(* Logix 5000 Routine export Unit1_Hold; software revision 20.05 *)

TYPE Unit_Type :   // Common information for a unit
STRUCT
   Alm_Reset : BOOL;   // Alarm reset
   Local : BOOL;   // Local/remote control indication
   Maint : BOOL;   // Maintenance privilege for device control
   Man_StartOpen : BOOL;   // Manual start/open from operator
   Man_StopClose : BOOL;   // Manual stop/close from operator
   Man_DevNum : DINT;   // Number of device started/stopped at OI
   Msg : DINT;   // Message number
   Time_Remaining : DINT;   // Remaining time in timed steps
END_STRUCT
END_TYPE

TYPE Seq_Type :   // Sequence Information
STRUCT
   Step_Num : DINT;   // Current step number
   Running : BOOL;   // Running indication
   PC_Start : BOOL;   // Sequence start request from PC
   LTP_Start : BOOL;   // Sequence start request from LTP
   Ons : BOOL;   // One-shot storage to start
   Auto_Start : BOOL;   // Auto-start request
   Auto_Ons : BOOL;   // Auto-start one-shot storage
   Req_Tmr : TIMER;   // Auto-start hold timer
END_STRUCT
END_TYPE

VAR_GLOBAL   (* controller tags *)
   Unit1_Hold : Seq_Type := (Req_Tmr.PRE := 5000);   // Unit Desc1 Hold Sequence
   Unit1_Sample : Seq_Type := (Req_Tmr.PRE := 5000);   // Unit Desc1 Sample Sequence
   Unit1 : Unit_Type;   // Unit Desc1
   Unit1_Shutdown : Seq_Type := (Req_Tmr.PRE := 5000);   // Unit Desc1 Shutdown Sequence
   Unit1_Eshutdown : Seq_Type := (Req_Tmr.PRE := 5000);   // Unit Desc1 E-Shutdown Sequence
END_VAR

PROGRAM MainProgram

ROUTINE Unit1_Hold   (* ladder *)
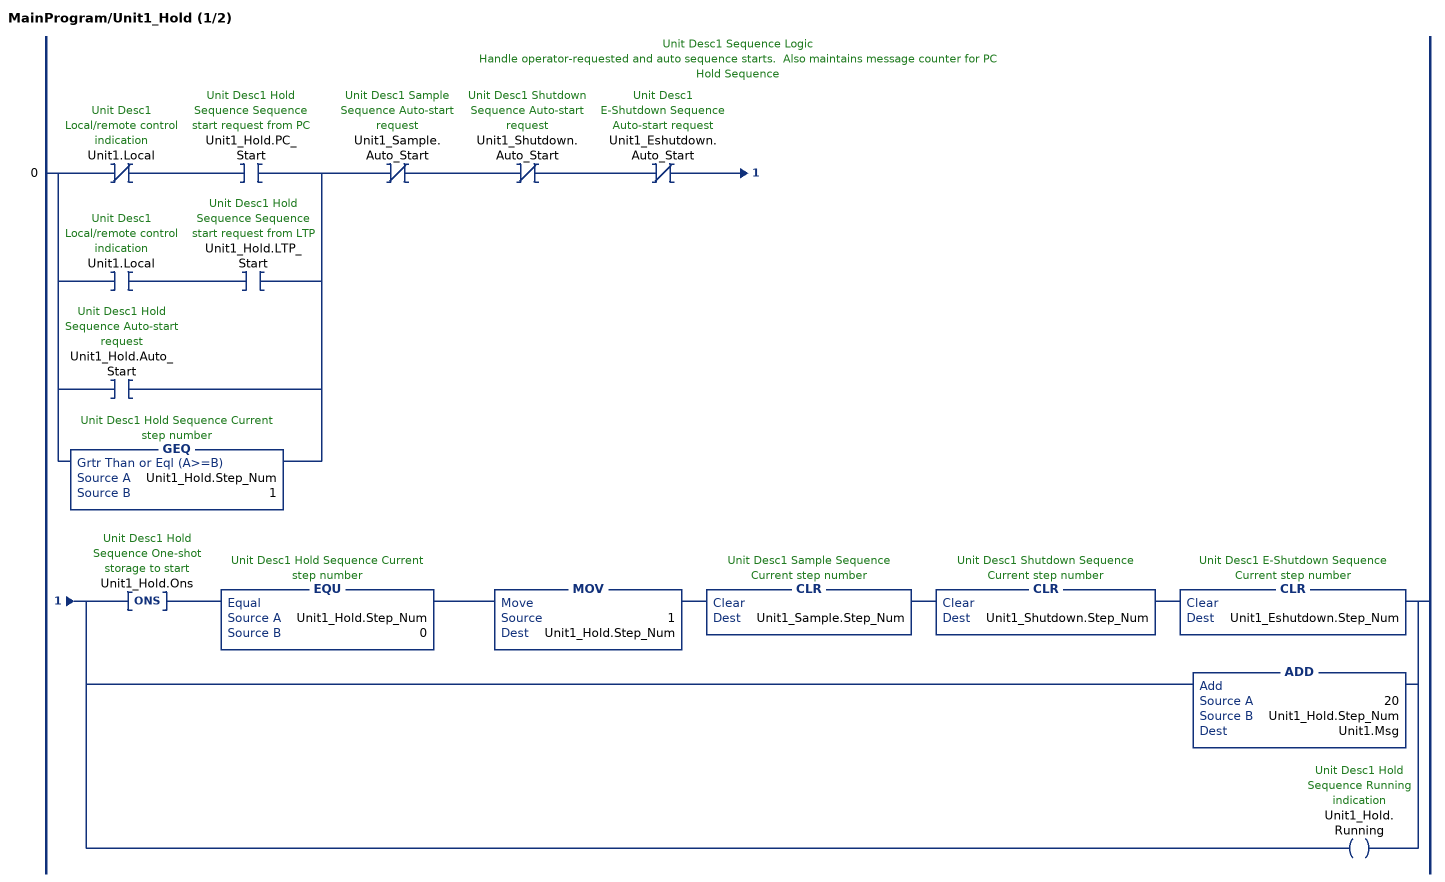
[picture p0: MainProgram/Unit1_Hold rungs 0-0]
   // Unit Desc1 Sequence Logic
   // Handle operator-requested and auto sequence starts.  Also maintains message counter for PC
   // Hold Sequence
   0: [XIO(Unit1.Local) XIC(Unit1_Hold.PC_Start) ,XIC(Unit1.Local) XIC(Unit1_Hold.LTP_Start) ,XIC(Unit1_Hold.Auto_Start) ,GEQ(Unit1_Hold.Step_Num,1) ]XIO(Unit1_Sample.Auto_Start)XIO(Unit1_Shutdown.Auto_Start)XIO(Unit1_Eshutdown.Auto_Start)[ONS(Unit1_Hold.Ons) EQU(Unit1_Hold.Step_Num,0) MOV(1,Unit1_Hold.Step_Num) CLR(Unit1_Sample.Step_Num) CLR(Unit1_Shutdown.Step_Num) CLR(Unit1_Eshutdown.Step_Num) ,ADD(20,Unit1_Hold.Step_Num,Unit1.Msg) ,OTE(Unit1_Hold.Running) ];
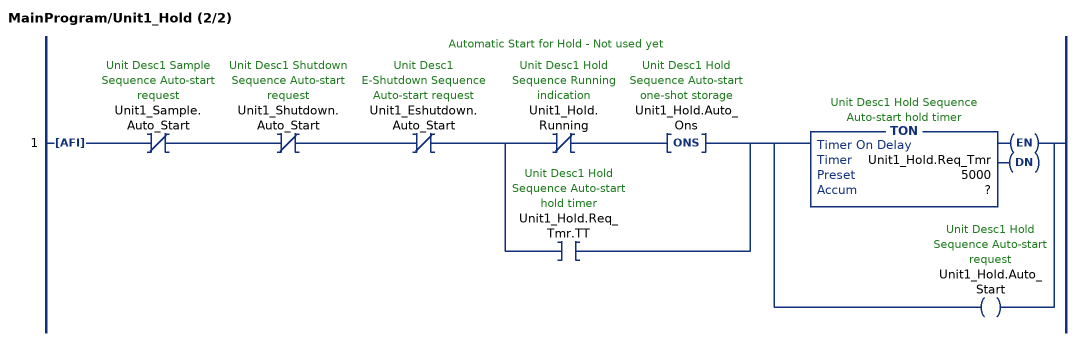
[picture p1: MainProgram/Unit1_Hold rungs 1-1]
   // Automatic Start for Hold - Not used yet
   1: AFI()XIO(Unit1_Sample.Auto_Start)XIO(Unit1_Shutdown.Auto_Start)XIO(Unit1_Eshutdown.Auto_Start)[XIO(Unit1_Hold.Running) ONS(Unit1_Hold.Auto_Ons) ,XIC(Unit1_Hold.Req_Tmr.TT) ][TON(Unit1_Hold.Req_Tmr,?,?) ,OTE(Unit1_Hold.Auto_Start) ];
END_ROUTINE
END_PROGRAM
